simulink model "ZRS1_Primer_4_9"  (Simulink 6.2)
settings: Solver=ode45  StartTime=0.0  StopTime=10.0  FixedStep=1.e-5  RelTol=1.e-3
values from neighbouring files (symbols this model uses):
  kp = 19    [ZRS1_Primer4_9.m]    (also in ZRS1_Primer4_10_1.m = 18; ZRS1_Primer4_10_2.m = 18; ZRS1_Primer4_10_nih_preiz.m = 30)
  motnja = 1    [ZRS1_Primer4_9.m]
  referenca = 0    [ZRS1_Primer4_9.m]    (also in ZRS1_Primer4_10_1.m = 1; ZRS1_Primer4_10_2.m = 1; ZRS1_Primer4_10_nih_preiz.m = 1)
  td = 4/19    (= 0.210526315789)    [ZRS1_Primer4_9.m]    (also in ZRS1_Primer4_10_1.m = 0.351; ZRS1_Primer4_10_2.m = 0.7692; ZRS1_Primer4_10_nih_preiz.m = 0)
  ti = 2    [ZRS1_Primer4_9.m]    (also in ZRS1_Primer4_10_1.m = 1.405; ZRS1_Primer4_10_2.m = 3.077; ZRS1_Primer4_10_nih_preiz.m = inf)

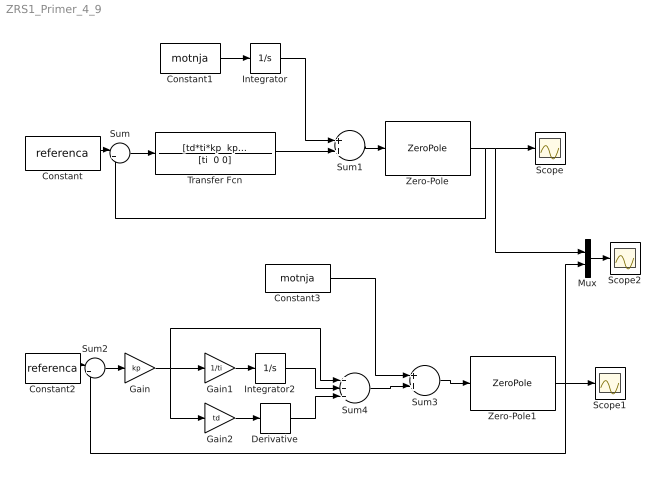
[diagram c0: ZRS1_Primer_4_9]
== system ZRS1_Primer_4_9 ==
  Constant : Constant  Value=referenca
  Constant1 : Constant  Value=motnja
  Constant2 : Constant  Value=referenca
  Constant3 : Constant  Value=motnja
  Derivative : Derivative
  Gain : Gain  Gain=kp
  Gain1 : Gain  Gain=1/ti
  Gain2 : Gain  Gain=td
  Integrator : Integrator
  Integrator2 : Integrator
  Mux : Mux  Inputs=2
  Scope : Scope
  Scope1 : Scope
  Scope2 : Scope
  Sum : Sum  Inputs=|+-
  Sum1 : Sum
  Sum2 : Sum  Inputs=|+-
  Sum3 : Sum
  Sum4 : Sum  Inputs=+++
  Transfer Fcn : TransferFcn  Numerator="[td*ti*kp  kp*ti  kp  ]"  Denominator="[ti  0 0]"
  Zero-Pole : ZeroPole  Zeros=[0]  Poles="[-1  -1/5]"  Gain=1/5
  Zero-Pole1 : ZeroPole  Zeros=[]  Poles="[-1  -1/5]"  Gain=1/5
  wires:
  Constant/1 -> Sum/1
  Sum/1 -> Transfer Fcn/1
  Transfer Fcn/1 -> Sum1/2
  Sum1/1 -> Zero-Pole/1
  Zero-Pole/1 -> Sum/2, Scope/1, Mux/1
  Constant1/1 -> Integrator/1
  Integrator/1 -> Sum1/1
  Constant2/1 -> Sum2/1
  Sum2/1 -> Gain/1
  Sum3/1 -> Zero-Pole1/1
  Zero-Pole1/1 -> Sum2/2, Scope1/1, Mux/2
  Constant3/1 -> Sum3/1
  Gain/1 -> Gain1/1, Sum4/1, Gain2/1
  Gain1/1 -> Integrator2/1
  Integrator2/1 -> Sum4/2
  Gain2/1 -> Derivative/1
  Derivative/1 -> Sum4/3
  Sum4/1 -> Sum3/2
  Mux/1 -> Scope2/1
